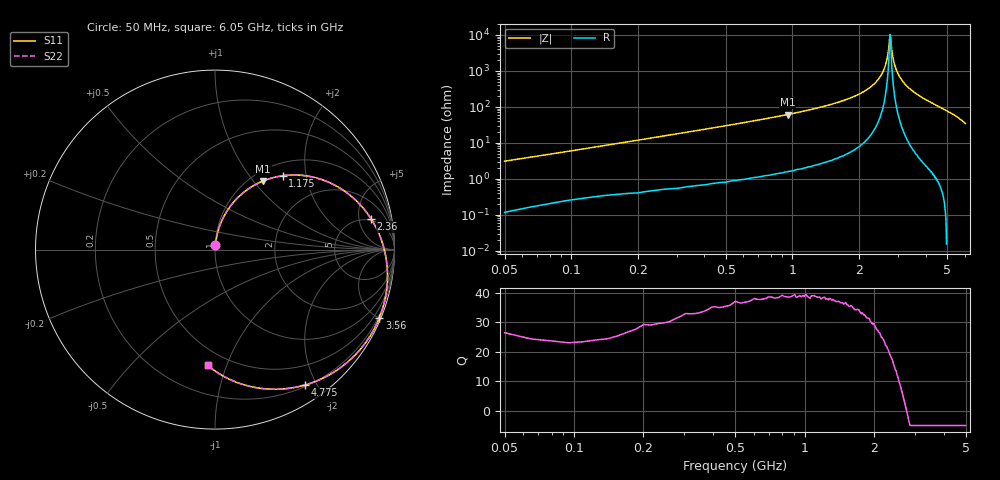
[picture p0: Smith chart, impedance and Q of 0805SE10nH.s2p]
! AVX Thin Film Operation		Date: May 2002
! Description: Accu-L® Series, Thin Film, SMD, RF Inductors
! Part Number: L0805100GEWTR
! 50 MHz  -  6.05 GHz
! Serial Measurements
# mhz S db R 50
!	S11		S21		S12		S22
!	dB	Phase	dB	Phase	dB	Phase	dB	Phase
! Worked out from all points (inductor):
!   401 points, 50 MHz to 6.05 GHz, reference 50 ohm
!   read as 1/Y11, port 2 shorted: L = 9.48 nH near 80 MHz
!   highest Q = 39 at 950 MHz (marker M1), where L = 10.3 nH
!   self-resonance near 2.75 GHz
!   S11 on the Smith chart (normalised r, x): 50 MHz: 1.00, +0.06; 1.175 GHz: 1.23, +1.47; 2.36 GHz: 4.62, +7.39; 3.56 GHz: 0.11, -5.02; 4.775 GHz: 0.22, -1.85; 6.05 GHz: 0.39, -0.86
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50  -30.90 85.1  -0.01 -1.9  -0.01 -1.9  -30.90 85.1
170  -20.75 81.4  -0.07 -6.2  -0.07 -6.2  -20.75 81.4
320  -15.42 76.5  -0.17 -11.5  -0.17 -11.5  -15.42 76.5
575  -10.57 67.8  -0.47 -20.4  -0.47 -20.4  -10.57 67.8
950  -6.63 55.0  -1.16 -33.0  -1.16 -33.0  -6.63 55.0
1055  -5.85 51.5  -1.42 -36.4  -1.42 -36.4  -5.85 51.5
1175  -5.08 47.6  -1.74 -40.3  -1.74 -40.3  -5.08 47.6
2060  -1.66 20.0  -5.26 -67.1  -5.26 -67.1  -1.66 20.0
2360  -1.05 11.2  -7.09 -75.4  -7.09 -75.4  -1.05 11.2
3050  -0.25 -8.4  -14.12 -93.0  -14.10 -93.0  -0.25 -8.4
3245  -0.15 -13.8  -17.92 -96.9  -17.90 -96.9  -0.15 -13.8
3395  -0.10 -18.0  -22.68 -98.3  -22.70 -98.3  -0.10 -18.0
3485  -0.08 -20.4  -27.60 -95.3  -27.60 -95.3  -0.08 -20.4
3560  -0.07 -22.5  -34.28 -49.3  -34.30 -49.3  -0.07 -22.5
3605  -0.07 -23.7  -40.09 -15.3  -40.00 -15.3  -0.07 -23.7
3695  -0.08 -26.2  -29.10 51.2  -29.10 51.2  -0.08 -26.2
3785  -0.09 -28.7  -23.58 57.9  -23.60 57.9  -0.09 -28.7
4055  -0.19 -36.2  -15.89 55.3  -15.90 55.3  -0.19 -36.2
4385  -0.42 -45.4  -11.26 47.8  -11.30 47.8  -0.42 -45.4
4775  -0.86 -56.3  -7.92 38.1  -7.92 38.1  -0.86 -56.3
5060  -1.30 -64.5  -6.19 30.9  -6.19 30.9  -1.30 -64.5
6050  -3.78 -93.6  -2.52 5.5  -2.52 5.5  -3.78 -93.6
